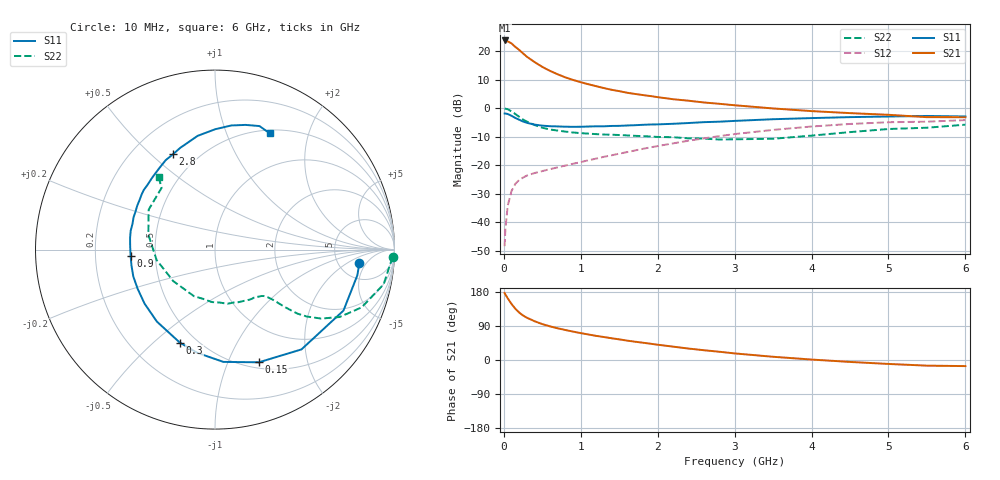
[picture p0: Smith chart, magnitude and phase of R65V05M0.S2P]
! SIEMENS Small Signal Semiconductors
! BFR193
! Si NPN RF Bipolar Junction Transistor in SOT23
! VCE = 5 V  IC = 5 mA
! Common Emitter S-Parameters:  May  1996
# GHz  S  MA  R  50
!  f  S11  S21  S12  S22
! GHz  MAG  ANG  MAG  ANG  MAG  ANG  MAG  ANG
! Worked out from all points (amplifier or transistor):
!   36 points, 10 MHz to 6 GHz, reference 50 ohm
!   highest |S21| = 23.8 dB at 10 MHz (marker M1)
!   |S21| within 3 dB of that: start of sweep to 184.3 MHz
!   unconditionally stable (mu >= 1): 904.8 MHz to 2.016 GHz
!   at 250 MHz: K = 0.43, MSG = 21.8 dB, |S12| = -24.3 dB
!   at 1.4 GHz: K = 1.06, MAG = 10.0 dB, |S12| = -16.5 dB
!   at 6 GHz: K = 0.96, MSG = 0.5 dB, |S12| = -4.2 dB
!   lowest NFmin = 1.20 dB at 450 MHz
!   S11 on the Smith chart (normalised r, x): 10 MHz: 7.88, -3.45; 150 MHz: 0.57, -1.30; 300 MHz: 0.41, -0.61; 900 MHz: 0.36, -0.03; 2.8 GHz: 0.37, +0.59; 6 GHz: 0.54, +1.44
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0.01  0.8079 -5.4  15.44 176.8  0.0038 85.2  0.9908 -2.4
0.02  0.8058 -10.3  15.18 172.9  0.0075 85.3  0.9798 -4.7
0.05  0.7923 -25.4  14.87 162.9  0.0194 76.7  0.9593 -11.6
0.1  0.7357 -49.1  13.69 147.8  0.0353 66.7  0.8783 -21.5
0.15  0.6739 -68.7  11.87 135.0  0.0472 59.2  0.7896 -28.4
0.2  0.6275 -85.7  10.53 125.2  0.0553 53.9  0.7056 -33.0
0.25  0.5837 -99.7  9.151 117.4  0.0607 50.6  0.6327 -36.1
0.3  0.5541 -110.7  7.998 111.5  0.0658 48.9  0.5825 -37.8
0.4  0.5155 -128.9  6.439 102.3  0.073 47.2  0.5068 -39.4
0.5  0.4946 -142.5  5.303 94.7  0.0789 47.9  0.4541 -40.3
0.6  0.4833 -152.9  4.52 88.8  0.0854 49.1  0.4235 -41.0
0.7  0.4792 -161.8  3.936 83.6  0.0918 50.2  0.4046 -41.7
0.9  0.4714 -175.8  3.134 74.9  0.1061 53.3  0.3751 -43.6
1.1  0.4774 172.4  2.631 67.3  0.1221 56.3  0.3581 -47.0
1.3  0.4814 162.9  2.256 60.6  0.1403 58.0  0.3452 -50.7
1.6  0.4975 150.6  1.87 51.2  0.1696 59.3  0.3334 -58.1
2.2  0.5331 130.7  1.438 35.3  0.2417 57.7  0.3098 -76.9
2.8  0.5803 113.8  1.196 21.8  0.3237 51.4  0.2823 -103.6
3.5  0.641 98.7  0.99 8.5  0.4165 41.1  0.2912 -142.8
4.5  0.6976 82.5  0.82 -5.1  0.5293 24.2  0.3808 167.3
5.5  0.7315 70.2  0.697 -14.9  0.5803 7.1  0.4546 130.9
6  0.7162 64.8  0.695 -16.1  0.6184 2.1  0.5142 127.7
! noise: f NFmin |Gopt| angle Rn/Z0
0.45  1.2  0.26  102  0.14
0.9  1.25  0.38  145  0.12
1.8  2.05  0.56  -161  0.12
